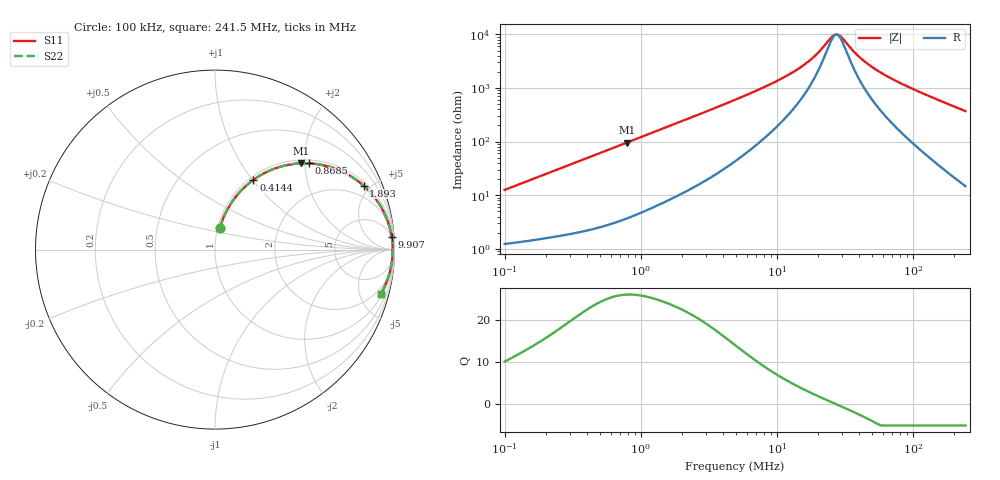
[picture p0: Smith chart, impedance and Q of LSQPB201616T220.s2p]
! LSQPB201616T220  S-PARAMETER MODEL  ( General Type )
! Model Generated by TAIYO YUDEN Corporation (http://www.ty-top.com)
! Version 2.0
! TAIYO YUDEN Control No. 100810NC14SB-FKC
! Copyright(c) 2008 TAIYO YUDEN CO.,LTD. All Rights Reserved.
! Product Description (link to TY-COMPAS)
! https://ds.yuden.co.jp/TYCOMPAS/or/detail?pn=LSQPB201616T220K&u=M
! Products Name : Inductors
! Characteristics :
!  Inductance : 22 uH , SRF(min) : 24 MHz , DC Resistance(max) : 1.3 Ohm
!  Rated Current : Saturation :310 mA , Temp Rise : 310 mA (40 degC)
!  Case Size : 2.0 x 1.6 / 0.079 x 0.063 [mm/inch] , Thickness : 1.6 / 0.063 [mm/inch]
!  (Conditions: Temperature = 25 degC , DC Bias Current/Voltage = 0A / 0V)
! External Node Assignments :
!  1  o---GGG---o  2
! GND o---------o GND
! Frequency Range : 0.1MHz  -  241.513628MHz  [ 402 STEP ]
# MHz S RI R 50
! Freq[MHz].  S11 Real  S11 Imag  S21 Real  S21 Imag  S12 Real  S12 Imag  S22 Real  S22 Imag
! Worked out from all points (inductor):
!   401 points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, 100 kHz to 241.5 MHz, reference 50 ohm
!   read as one part in series: L = 19.8 uH near 104 kHz
!   highest Q = 26 at 787.9 kHz (marker M1), where L = 19.3 uH
!   self-resonance near 27.27 MHz
!   S11 on the Smith chart (normalised r, x): 100 kHz: 1.02, +0.25; 414.4 kHz: 1.04, +1.01; 868.5 kHz: 1.08, +2.10; 1.893 MHz: 1.20, +4.55; 9.907 MHz: 5, +27; 241.5 MHz: 1.29, -7.41
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0.1  0.027 0.12  0.973 -0.12  0.973 -0.12  0.027 0.12
0.209594  0.0756 0.2352  0.9244 -0.2352  0.9244 -0.2352  0.0756 0.2352
0.368674  0.1803 0.362  0.8197 -0.362  0.8197 -0.362  0.1803 0.362
0.414369  0.2143 0.3889  0.7857 -0.3889  0.7857 -0.3889  0.2143 0.3889
0.588328  0.3449 0.4559  0.6551 -0.4559  0.6551 -0.4559  0.3449 0.4559
0.787915  0.4784 0.4807  0.5216 -0.4807  0.5216 -0.4807  0.4784 0.4807
0.868493  0.5248 0.4805  0.4752 -0.4805  0.4752 -0.4805  0.5248 0.4805
1.359207  0.7209 0.4288  0.2791 -0.4288  0.2791 -0.4288  0.7209 0.4288
1.892607  0.8277 0.3564  0.1723 -0.3564  0.1723 -0.3564  0.8277 0.3564
2.90484  0.9132 0.257  0.0868 -0.257  0.0868 -0.257  0.9132 0.257
4.914404  0.9625 0.1577  0.0375 -0.1577  0.0375 -0.1577  0.9625 0.1577
9.90685  0.9844 0.072  0.0156 -0.072  0.0156 -0.072  0.9844 0.072
14.06591  0.988 0.0431  0.012 -0.0431  0.012 -0.0431  0.988 0.0431
18.11814  0.9893 0.0256  0.0107 -0.0256  0.0107 -0.0256  0.9893 0.0256
25.22833  0.99 0.00483  0.00997 -0.00483  0.00997 -0.00483  0.99 0.00483
27.80836  0.9901 -0.00107  0.00994 0.00107  0.00994 0.00107  0.9901 -0.00107
30.06109  0.99 -0.00579  0.00996 0.00579  0.00996 0.00579  0.99 -0.00579
37.24223  0.9897 -0.0191  0.0103 0.0191  0.0103 0.0191  0.9897 -0.0191
43.52056  0.9892 -0.0292  0.0108 0.0292  0.0108 0.0292  0.9892 -0.0292
66.79689  0.9862 -0.0614  0.0138 0.0614  0.0138 0.0614  0.9862 -0.0614
117.495  0.9749 -0.1213  0.0251 0.1213  0.0251 0.1213  0.9749 -0.1213
241.5136  0.9237 -0.2464  0.0763 0.2464  0.0763 0.2464  0.9237 -0.2464
